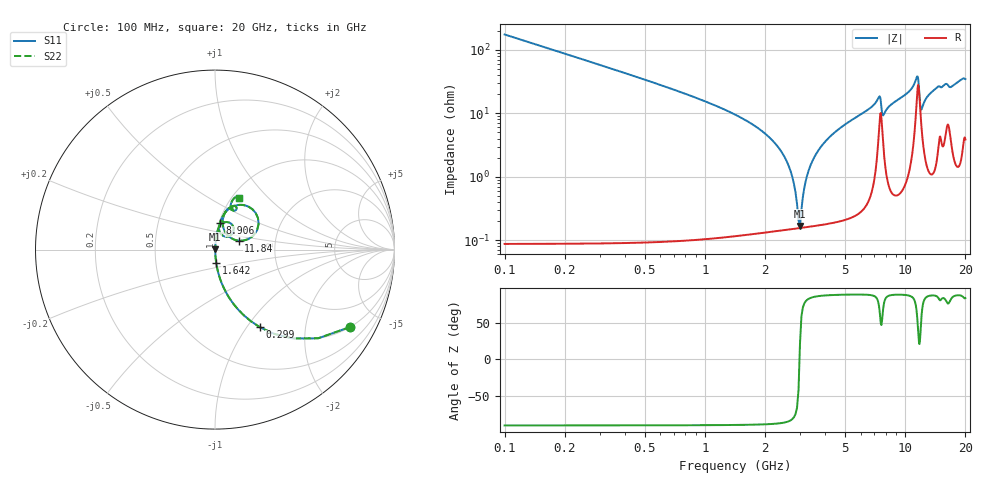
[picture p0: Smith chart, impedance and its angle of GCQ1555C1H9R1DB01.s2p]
!Murata Part Number: GCQ1555C1H9R1DB01
!These Parameters are Measured in Series Mode Connection
!Data Generated on Jan 08, 2026
!  o--ll--o
!Port1  Port2
!  o------o
!Operation Temp=25[degC], DC Bias Voltage=0[V]
!Freq. Start=100[MHz] Stop=20[GHz] 401[Steps]
# Hz S RI R 50
!Freq.(Hz) S11(Real) S11(Imag) S21(Real) S21(Imag) S12(Real) S12(Imag) S22(Real) S22(Imag)
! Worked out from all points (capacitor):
!   401 points, 100 MHz to 20 GHz, reference 50 ohm
!   read as one part in series: C = 9.1 pF near 199.5 MHz
!   lowest |Z| = 167 mohm at 2.986 GHz (marker M1)
!   series resonance near 2.97 GHz, so ESL is about 320 pH
!   S11 on the Smith chart (normalised r, x): 100 MHz: 1.00, -3.49; 299 MHz: 1.00, -1.16; 1.642 GHz: 1.00, -0.15; 8.906 GHz: 1.01, +0.31; 11.84 GHz: 1.30, +0.13; 20 GHz: 1.08, +0.69
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1e8  0.7531 -0.431  0.2469 0.431  0.2469 0.431  0.7531 -0.431
2.99e8  0.2514 -0.433  0.7486 0.433  0.7486 0.433  0.2514 -0.433
6.4725e8  0.0629 -0.2409  0.9371 0.2409  0.9371 0.2409  0.0629 -0.2409
1.64225e9  0.00664 -0.0734  0.9934 0.0734  0.9934 0.0734  0.00664 -0.0734
2.488e9  0.00188 -0.021  0.9981 0.021  0.9981 0.021  0.00188 -0.021
2.687e9  0.00163 -0.0118  0.9984 0.0118  0.9984 0.0118  0.00163 -0.0118
2.886e9  0.00154 -0.0034  0.9985 0.0034  0.9985 0.0034  0.00154 -0.0034
2.9855e9  0.00156 0.000605  0.9984 -0.000605  0.9984 -0.000605  0.00156 0.000605
3.23425e9  0.00171 0.0101  0.9983 -0.0101  0.9983 -0.0101  0.00171 0.0101
3.43325e9  0.00195 0.0172  0.998 -0.0172  0.998 -0.0172  0.00195 0.0172
4.478e9  0.00447 0.0506  0.9955 -0.0506  0.9955 -0.0506  0.00447 0.0506
6.7665e9  0.0203 0.1213  0.9797 -0.1213  0.9797 -0.1213  0.0203 0.1213
7.41325e9  0.0787 0.1512  0.9213 -0.1512  0.9213 -0.1512  0.0787 0.1512
7.7615e9  0.0404 0.0796  0.9596 -0.0796  0.9596 -0.0796  0.0404 0.0796
8.90575e9  0.0275 0.1477  0.9725 -0.1477  0.9725 -0.1477  0.0275 0.1477
1.005e10  0.0446 0.1879  0.9554 -0.1879  0.9554 -0.1879  0.0446 0.1879
1.1443e10  0.2078 0.2255  0.7922 -0.2255  0.7922 -0.2255  0.2078 0.2255
1.1841e10  0.1316 0.0495  0.8684 -0.0495  0.8684 -0.0495  0.1316 0.0495
1.204e10  0.07 0.0808  0.93 -0.0808  0.93 -0.0808  0.07 0.0808
1.338325e10  0.0507 0.1944  0.9493 -0.1944  0.9493 -0.1944  0.0507 0.1944
1.67165e10  0.0997 0.2181  0.9003 -0.2181  0.9003 -0.2181  0.0997 0.2181
2e10  0.1322 0.287  0.8678 -0.287  0.8678 -0.287  0.1322 0.287
